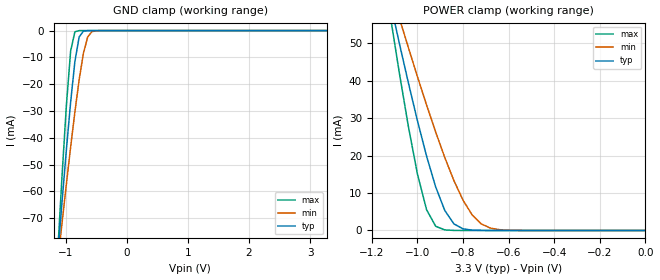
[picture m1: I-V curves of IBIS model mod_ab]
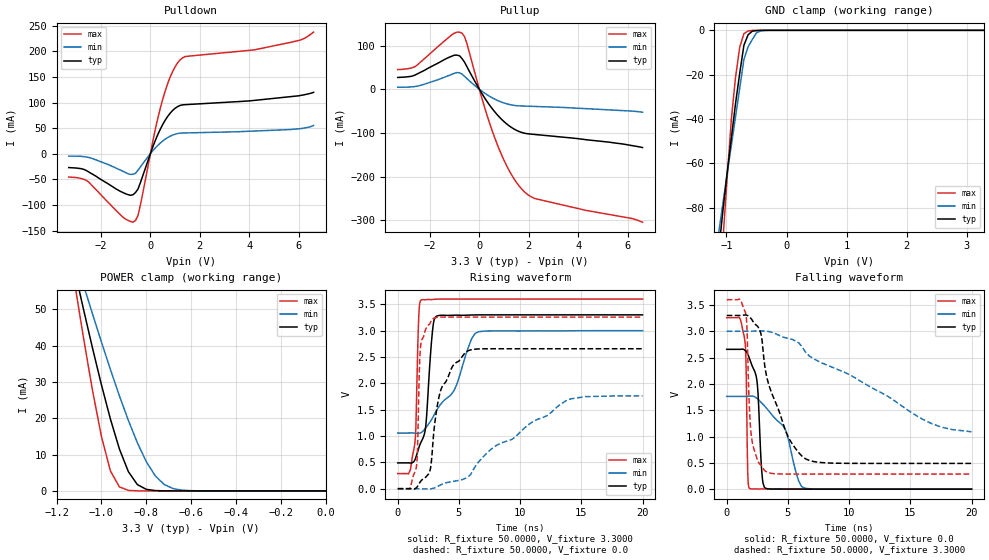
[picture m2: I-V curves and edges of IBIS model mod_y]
| IBIS (I/O, Buffer, Information, Specification) Model, officially
| electronic behavioral standard for Buffer structures of digital pins.
[IBIS ver]  4.0
[File name] 54ac08_3v3_rev1.ibs
[File Rev]  1.0
[Date]   28 June 2016
[Source]   CAD & Design Services (Catania) - STMicroelectronics
[Notes]
  (Note1) This IBIS model is the model of the product with package
   (Flat14 package elements);
  (Note2) This IBIS model is extracted with nominal 3.3V power supply
   (min:3.0V, typ:3.3V, max:3.6V);
  (Note3) This model has few Warnings about the non-monotonicity
   of I-V curves, but they are not indicative of problems
   inside the model;
[Copyright] (c) 2016 STMicroelectronics
|   Component 54AC08
[Component] 54AC08
[Manufacturer] STMicroelectronics
[Package]
| variable   typ   min   max
R_pkg   0.0   0.0   0.0
L_pkg   0.0H   0.0H   0.0H
C_pkg   0.0F   0.0F   0.0F
[Pin]  signal_name   model_name   R_pin   L_pin   C_pin
1   1A   mod_ab   179.4m   5.61nH   1.01pF
2   1B   mod_ab   114.3m   3.16nH   0.80pF
3   1Y   mod_y   120.1m   3.55nH   1.04pF
4   2A   mod_ab   99.9m   2.85nH   1.04pF
5   2B   mod_ab   116.9m   3.35nH   1.04pF
6   2Y   mod_y   143.6m   4.16nH   0.80pF
7   GND   GND   172.3m   5.41nH   1.01pF
8   3Y   mod_y   179.4m   5.61nH   1.01pF
9   3A   mod_ab   155.5m   4.66nH   0.80pF
10   3B   mod_ab   116.9m   3.35nH   1.04pF
11   4Y   mod_y   94.7m   2.65nH   1.04pF
12   4A   mod_ab   113.3m   3.25nH   1.04pF
13   4B   mod_ab   145.2m   4.26nH   0.80pF
14   VCC   POWER   172.3m   5.41nH   1.01pF
| Models and submodels in the file (2): mod_ab (Input), mod_y (I/O)
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|   Model mod_ab
[Model]   mod_ab
Model_type Input
Vinl   =   1.000V
Vinh   =   2.300V
C_comp   0.584pF   0.423pF   0.702pF
[Temperature Range]  25.0000   0.1250k   -55.0000
[Voltage Range]   3.3000V   3.0000V   3.6000V
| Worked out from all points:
|   GND clamp passes 1 mA (typ) near -0.74 V on its own axis
|   POWER clamp passes 1 mA (typ) near -0.82 V on its own axis
[GND_clamp]
|Voltage   I(typ)   I(min)   I(max)
-3.3V     -749mA     -568.4mA   -1.036A
-1.13V    -83.59mA   -86.25mA   -82mA
-1.06V    -63.75mA   -71.67mA   -54.05mA
-990mV    -44.61mA   -57.39mA   -28.12mA
-920mV    -26.72mA   -43.53mA   -7.666mA
-850mV    -11.52mA   -30.35mA   -438.9uA
-780mV    -2.357mA   -18.3mA    -11.16uA
-710mV    -202.6uA   -8.405mA   -269.9nA
-640mV    -13.61uA   -2.367mA   -6.525nA
-570mV    -893.7nA   -396.6uA   -166.8pA
-430mV    -3.851nA   -7.049uA   -9.012pA
3.28V     6.52pA     5.985nA    5.92pA
[POWER_clamp]
|Voltage   I(typ)   I(min)   I(max)
-3.28V    721.1mA    542.9mA    1.005A
-1.12V    61.08mA    64.91mA    57.6mA
-1.08V    50.1mA     56.8mA     42.24mA
-1.04V    39.44mA    48.83mA    27.8mA
-1V       29.27mA    41.04mA    15.03mA
-960mV    19.83mA    33.48mA    5.531mA
-920mV    11.6mA     26.24mA    1.117mA
-880mV    5.324mA    19.45mA    149.5uA
-840mV    1.752mA    13.29mA    18.09uA
-760mV    95.86uA    4.148mA    257.2nA
-680mV    4.309uA    633uA      3.657nA
0V        6.6pA      45.39pA    7.2pA
|   Model mod_y
[Model]   mod_y
Model_type I/O
Polarity   Non-Inverting
Vinl   =   1.000V
Vinh   =   2.300V
Vmeas  =   1.650V
Cref   =   50pF
Rref   =   500
C_comp   3.207pF   2.433pF   4.228pF
[Temperature Range]  25.0000   0.1250k   -55.0000
[Voltage Range]   3.3000V   3.0000V   3.6000V
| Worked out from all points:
|   slope of the pulldown table from 0 to 0.495 V, typ, clamps not added: 8.73 ohm
|   slope of the pullup table from 0 to 0.495 V, typ, clamps not added: 11.6 ohm
|   GND clamp passes 1 mA (typ) near -0.60 V on its own axis
|   POWER clamp passes 1 mA (typ) near -0.82 V on its own axis
|   rising waveform, R_fixture 50.0000, V_fixture 3.3000: 20-80 % time 548ps typ, 2.59ns min, 233ps max; typ from 0.489 V to 3.3 V
|   rising waveform, R_fixture 50.0000, V_fixture 0.0: 20-80 % time 1.37ns typ, 6.2ns min, 230ps max; typ from 0 V to 2.66 V
|   falling waveform, R_fixture 50.0000, V_fixture 0.0: 20-80 % time 384ps typ, 1.92ns min, 140ps max; typ from 2.66 V to 0 V
|   falling waveform, R_fixture 50.0000, V_fixture 3.3000: 20-80 % time 1.98ns typ, 8.59ns min, 376ps max; typ from 3.3 V to 0.489 V
[Pulldown]
|Voltage   I(typ)   I(min)   I(max)
-3.3V     -27.02mA   -4.701mA   -45.61mA
-2.6V     -32.52mA   -6.315mA   -51.73mA
-1.1V     -76.02mA   -34.53mA   -124.4mA
-700mV    -80.04mA   -40.16mA   -133.7mA
-500mV    -68.93mA   -32.08mA   -120.6mA
200mV     25.93mA    11.34mA    47.73mA
500mV     57.16mA    24.87mA    106.4mA
900mV     84.46mA    36.38mA    160.6mA
1.2V      94.2mA     40.13mA    183.1mA
1.4V      95.76mA    40.56mA    189.6mA
5.7V      111.6mA    47.42mA    217.8mA
6.6V      119.8mA    55.17mA    237.5mA
[Pullup]
|Voltage   I(typ)   I(min)   I(max)
-3.3V     27.02mA    4.701mA    45.04mA
-2.6V     32.52mA    6.315mA    51.73mA
-1V       78.22mA    36.94mA    128.8mA
-700mV    70.18mA    34.83mA    128.5mA
-600mV    62.24mA    29.61mA    120.7mA
-500mV    51.44mA    24.28mA    104.5mA
200mV     -18.57mA   -8.361mA   -39.23mA
700mV     -56.88mA   -24.76mA   -122.8mA
1.2V      -83.63mA   -34.73mA   -185.7mA
1.8V      -100.4mA   -38.51mA   -233.9mA
2.3V      -104mA     -39.52mA   -251.2mA
6.6V      -133.6mA   -52.67mA   -304.7mA
[GND_clamp]
|Voltage   I(typ)   I(min)   I(max)
-3.3V     -750.5mA   -569.2mA   -1.049A
-1.13V    -99.8mA    -91.54mA   -122.8mA
-1.06V    -81.6mA    -78.17mA   -95.14mA
-990mV    -64.61mA   -65.1mA    -67.22mA
-920mV    -48.9mA    -52.15mA   -40.51mA
-850mV    -33.2mA    -39.19mA   -21.39mA
-780mV    -19.49mA   -26.19mA   -7.724mA
-710mV    -6.761mA   -13.2mA    -1.514mA
-640mV    -2.019mA   -7.433mA   -302.5uA
-500mV    -143.5uA   -1.107mA   -6.459uA
-360mV    -6.928uA   -54.34uA   -66.17nA
3.28V     2.9pA      17.61pA    1.9pA
[POWER_clamp]
|Voltage   I(typ)   I(min)   I(max)
-3.28V    721.1mA    542.9mA    1.005A
-1.12V    61.08mA    64.91mA    57.6mA
-1.08V    50.1mA     56.8mA     42.24mA
-1.04V    39.44mA    48.83mA    27.8mA
-1V       29.27mA    41.04mA    15.03mA
-960mV    19.83mA    33.48mA    5.531mA
-920mV    11.6mA     26.24mA    1.117mA
-880mV    5.324mA    19.45mA    149.5uA
-840mV    1.752mA    13.29mA    18.09uA
-760mV    95.86uA    4.148mA    257.2nA
-680mV    4.309uA    633uA      3.657nA
0V        6.6pA      45.39pA    7.2pA
[Ramp]
| variable   typ   min   max
dV/dt_r  1.5940/1.4012n   1.0570/6.1928n   1.9543/0.3567n
dV/dt_f  1.6864/2.0337n   1.1649/8.7779n   1.9877/0.4851n
R_load = 50.0000
[Rising Waveform]
R_fixture= 50.0000
V_fixture= 3.3000
V_fixture_min= 3.0000
V_fixture_max= 3.6000
|time   V(typ)   V(min)   V(max)
0s        489.4mV    1.057V     286.6mV
880ps     489.6mV    1.057V     281.8mV
1.4ns     545.1mV    1.055V     861.8mV
1.72ns    772.4mV    1.052V     3.279V
1.88ns    871.9mV    1.061V     3.577V
2.28ns    1.171V     1.151V     3.589V
2.84ns    2.992V     1.344V     3.591V
3.22ns    3.281V     1.505V     3.598V
6.6ns     3.299V     2.979V     3.6V
20ns      3.3V       3V         3.6V
[Rising Waveform]
R_fixture= 50.0000
V_fixture= 0.0
V_fixture_min= 0.0
V_fixture_max= 0.0
|time   V(typ)   V(min)   V(max)
0s        132.2pV    0V         79.8pV
1.52ns    16.98mV    131.1uV    406mV
1.6ns     38.22mV    -186.6uV   628.7mV
1.88ns    141.6mV    -2.478mV   2.734V
2.64ns    349.9mV    -4.895mV   3.14V
2.92ns    1.004V     8.534mV    3.232V
3.52ns    1.875V     72.95mV    3.257V
5.72ns    2.616V     220.5mV    3.258V
13.74ns   2.657V     1.669V     3.258V
20ns      2.657V     1.762V     3.258V
[Falling Waveform]
R_fixture= 50.0000
V_fixture= 0.0
V_fixture_min= 0.0
V_fixture_max= 0.0
|time   V(typ)   V(min)   V(max)
0s        2.657V     1.762V     3.258V
1.44ns    2.648V     1.761V     2.896V
1.56ns    2.624V     1.762V     2.567V
1.72ns    2.567V     1.764V     310.4mV
1.9ns     2.459V     1.768V     8.794mV
2.48ns    2.043V     1.724V     4.179mV
2.86ns    353.7mV    1.638V     4.563mV
3.16ns    19.74mV    1.563V     3.086mV
6.36ns    1.648mV    19.8mV     1.478uV
20ns      -623nV     167.9uV    -14.61nV
[Falling Waveform]
R_fixture= 50.0000
V_fixture= 3.3000
V_fixture_min= 3.0000
V_fixture_max= 3.6000
|time   V(typ)   V(min)   V(max)
0s        3.3V       3V         3.6V
1.54ns    3.309V     3V         3.351V
1.64ns    3.305V     3V         3.151V
1.82ns    3.28V      2.999V     1.748V
2ns       3.238V     3V         1.04V
2.76ns    2.982V     3.006V     462.9mV
3.16ns    2.271V     3.003V     343.4mV
5.08ns    962mV      2.863V     287mV
6.48ns    571.9mV    2.589V     286.7mV
20ns      489.4mV    1.09V      286.6mV
